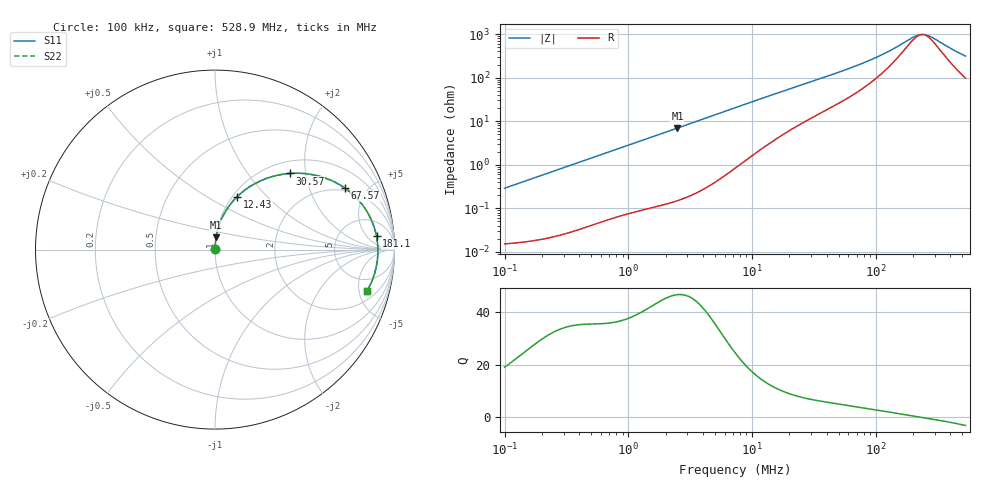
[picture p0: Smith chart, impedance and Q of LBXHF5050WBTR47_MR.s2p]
! LBXHF5050WBTR47_MR  S-PARAMETER MODEL  ( General Type )
! Model Generated by TAIYO YUDEN Corporation (http://www.ty-top.com)
! Version 1.0
! TAIYO YUDEN Control No. 210719NI43SB-FBB
! Copyright(c) 2021 TAIYO YUDEN CO.,LTD. All Rights Reserved.
! Product Description (link to TY-COMPAS)
! https://ds.yuden.co.jp/TYCOMPAS/or/detail?pn=LBXHF5050WBTR47NMR&u=M
! Products Name : Inductors
! Characteristics :
!  Inductance : 0.47 uH , SRF(min) : 180 MHz , DC Resistance(max) : 0.0144 Ohm
!  Rated Current : Saturation :6600 mA , Temp Rise : 3600 mA
!  Case Size : 5.0 x 5.0 / 0.197 x 0.197 [mm/inch] , Thickness : 2.2 / 0.087 [mm/inch]
!  (Conditions: Temperature = 25 degC , DC Bias Current/Voltage = 0A / 0V)
! External Node Assignments :
!  1  o---GGG---o  2
! GND o---------o GND
! Frequency Range : 0.1MHz  -  528.887669MHz  [ 402 STEP ]
# MHz S RI R 50
! Freq[MHz].  S11 Real  S11 Imag  S21 Real  S21 Imag  S12 Real  S12 Imag  S22 Real  S22 Imag
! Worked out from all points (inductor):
!   401 points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, 100 kHz to 528.9 MHz, reference 50 ohm
!   read as one part in series: L = 459 nH near 104.4 kHz
!   highest Q = 46.5 at 2.49 MHz (marker M1), where L = 444 nH
!   self-resonance near 236.8 MHz
!   S11 on the Smith chart (normalised r, x): 100 kHz: 1.00, +0.01; 12.43 MHz: 1.05, +0.69; 30.57 MHz: 1.24, +1.63; 67.57 MHz: 1.86, +3.55; 181.1 MHz: 12, +10; 528.9 MHz: 2.96, -5.96
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0.1  0.00016 0.00289  0.9998 -0.00289  0.9998 -0.00289  0.00016 0.00289
0.420401  0.000485 0.012  0.9995 -0.012  0.9995 -0.012  0.000485 0.012
1.767367  0.00355 0.0492  0.9964 -0.0492  0.9964 -0.0492  0.00355 0.0492
2.490355  0.00627 0.0689  0.9937 -0.0689  0.9937 -0.0689  0.00627 0.0689
4.4421  0.0182 0.1214  0.9818 -0.1214  0.9818 -0.1214  0.0182 0.1214
7.430023  0.049 0.196  0.951 -0.196  0.951 -0.196  0.049 0.196
12.42773  0.1241 0.2954  0.8759 -0.2954  0.8759 -0.2954  0.1241 0.2954
19.0792  0.2389 0.3761  0.7611 -0.3761  0.7611 -0.3761  0.2389 0.3761
24.15197  0.3223 0.4079  0.6777 -0.4079  0.6777 -0.4079  0.3223 0.4079
30.5735  0.4157 0.4243  0.5843 -0.4243  0.5843 -0.4243  0.4157 0.4243
44.96726  0.5753 0.4105  0.4247 -0.4105  0.4247 -0.4105  0.5753 0.4105
67.57036  0.725 0.3419  0.275 -0.3419  0.275 -0.3419  0.725 0.3419
95.21179  0.8169 0.2553  0.1831 -0.2553  0.1831 -0.2553  0.8169 0.2553
128.5312  0.8685 0.1712  0.1315 -0.1712  0.1315 -0.1712  0.8685 0.1712
181.1102  0.8998 0.0747  0.1002 -0.0747  0.1002 -0.0747  0.8998 0.0747
201.5975  0.9046 0.0448  0.0954 -0.0448  0.0954 -0.0448  0.9046 0.0448
219.6437  0.9068 0.0209  0.0932 -0.0209  0.0932 -0.0209  0.9068 0.0209
239.3053  0.9077 -0.00297  0.0923 0.00297  0.0923 0.00297  0.9077 -0.00297
255.1982  0.9075 -0.0209  0.0925 0.0209  0.0925 0.0209  0.9075 -0.0209
290.2204  0.9049 -0.057  0.0951 0.057  0.0951 0.057  0.9049 -0.057
436.1017  0.8744 -0.175  0.1256 0.175  0.1256 0.175  0.8744 -0.175
528.8877  0.8455 -0.2328  0.1545 0.2328  0.1545 0.2328  0.8455 -0.2328
